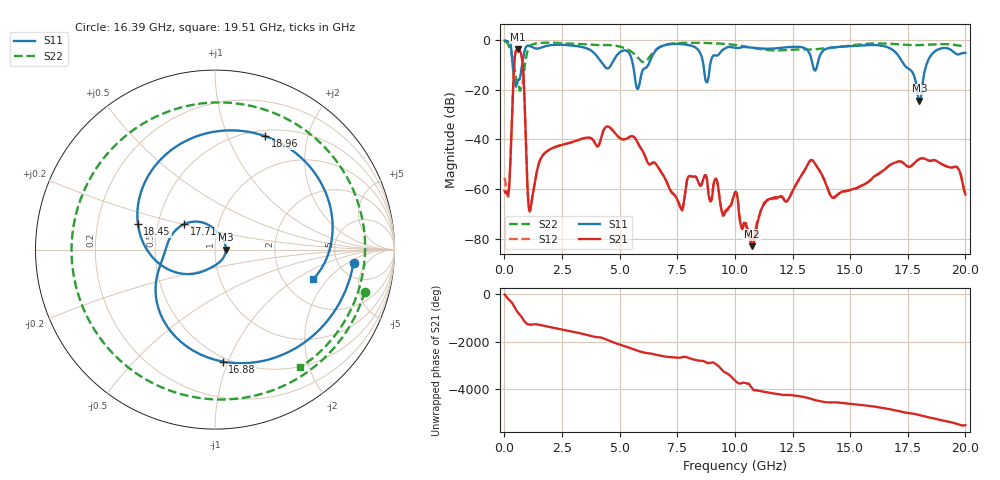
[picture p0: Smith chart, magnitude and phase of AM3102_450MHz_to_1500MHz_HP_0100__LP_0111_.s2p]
!Agilent Technologies,E8364B,MY43040894,A.07.50.67
!Agilent E8364B: A.07.50.67
!Date: Thursday, January 11, 2018 05:36:53
!Correction: S11(Full 2 Port(1,2))
!S21(Full 2 Port(1,2))
!S12(Full 2 Port(1,2))
!S22(Full 2 Port(1,2))
!S2P File: Measurements: S11, S21, S12, S22:
# Hz S  dB  R 50
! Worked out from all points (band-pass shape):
!   1601 points, 10 MHz to 20 GHz, reference 50 ohm
!   highest |S21| = -3.64 dB at 572.2 MHz (marker M1); lowest = -83.0 dB at 10.74 GHz (marker M2)
!   |S21| within 3 dB of the highest: 455.6 MHz to 752.7 MHz (297.1 MHz wide, 49.2 % of centre)
!   lowest |S11| = -24.3 dB at 18 GHz (marker M3), VSWR 1.13, Z = 56.5 + j0.0135 ohm
!   |S11| at or under -10 dB: 357.7 MHz to 764.6 MHz (406.9 MHz wide, 72.5 % of centre); 5.581 GHz to 6.236 GHz (655.1 MHz wide, 11.1 % of centre); 17.35 GHz to 18.31 GHz (951 MHz wide, 5.33 % of centre)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
!   |S22| runs from -20.3 to -0.4 dB; largest |S21 - S12| = 0.0018
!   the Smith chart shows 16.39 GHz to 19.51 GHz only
!   S11 on the Smith chart (normalised r, x): 16.39 GHz: 6.97, -2.52; 16.88 GHz: 0.47, -0.95; 17.71 GHz: 0.68, +0.20; 18.45 GHz: 0.39, +0.14; 18.96 GHz: 0.57, +1.38; 19.51 GHz: 2.88, -1.42
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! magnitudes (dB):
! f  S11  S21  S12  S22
! 10 MHz  -0.1  -60.9  -55.5  -0.4
! 197.4 MHz  -0.7  -60.4  -60.2  -2.6
! 572.2 MHz  -16.5  -3.6  -3.6  -17.0
! 784.6 MHz  -9.0  -8.8  -8.8  -17.3
! 1.109 GHz  -2.3  -69.1  -68.5  -2.3
! 3.346 GHz  -2.7  -39.8  -39.8  -1.5
! 5.782 GHz  -19.6  -41.2  -41.2  -6.9
! 6.682 GHz  -3.1  -51.4  -51.4  -3.0
! 7.669 GHz  -1.5  -68.0  -68.8  -1.1
! 10.01 GHz  -3.1  -61.5  -61.3  -1.9
! 10.74 GHz  -3.0  -83.0  -80.6  -3.0
! 13.34 GHz  -8.4  -48.3  -48.3  -3.8
! 14.27 GHz  -2.8  -63.6  -63.4  -3.0
! 16.39 GHz  -2.2  -52.8  -52.9  -1.2
! 16.68 GHz  -3.0  -50.7  -50.6  -1.3
! 16.88 GHz  -4.1  -49.6  -49.6  -1.5
! 17.71 GHz  -13.1  -50.3  -50.2  -1.9
! 18 GHz  -24.3  -47.9  -47.9  -1.9
! 18.45 GHz  -6.9  -48.7  -48.6  -1.8
! 18.96 GHz  -3.2  -49.9  -49.9  -1.5
! 19.51 GHz  -4.9  -51.1  -51.1  -1.8
! 20 GHz  -5.1  -62.2  -61.5  -2.5
